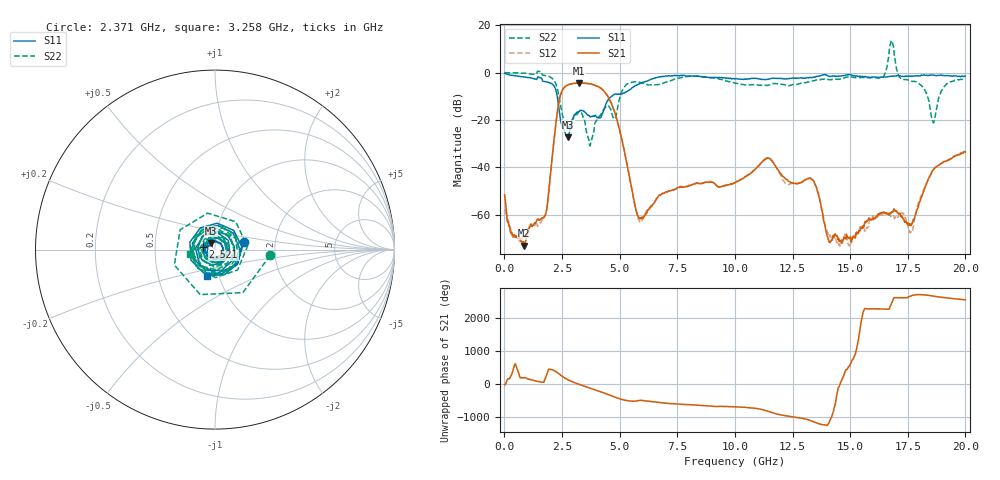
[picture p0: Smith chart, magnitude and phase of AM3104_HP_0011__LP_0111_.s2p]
!Created with skrf (http://scikit-rf.org).
# Hz S RI R 50.0
!freq ReS11 ImS11 ReS21 ImS21 ReS12 ImS12 ReS22 ImS22
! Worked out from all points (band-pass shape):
!   1601 points, 10 MHz to 20 GHz, reference 50 ohm
!   highest |S21| = -4.39 dB at 3.246 GHz (marker M1); lowest = -73.2 dB at 859.6 MHz (marker M2)
!   |S21| within 3 dB of the highest: 2.516 GHz to 4.278 GHz (1.762 GHz wide, 51.9 % of centre)
!   lowest |S11| = -27.3 dB at 2.746 GHz (marker M3), VSWR 1.09, Z = 47.7 + j3.49 ohm
!   |S11| at or under -10 dB: 2.293 GHz to 4.651 GHz (2.358 GHz wide, 67.9 % of centre)
!   |S22| runs from -31.0 to 13.6 dB; largest |S21 - S12| = 0.037
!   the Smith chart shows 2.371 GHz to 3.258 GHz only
!   S11 on the Smith chart (normalised r, x): 2.371 GHz: 1.38, +0.12; 2.521 GHz: 0.87, +0.02; 3.258 GHz: 0.88, -0.26
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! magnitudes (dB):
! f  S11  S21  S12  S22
! 10 MHz  -0.3  -51.7  -57.6  0.0
! 859.6 MHz  -1.9  -73.2  -69.1  -0.2
! 1.784 GHz  -3.8  -60.0  -60.2  -1.3
! 2.371 GHz  -15.6  -12.2  -12.2  -10.2
! 2.521 GHz  -23.3  -7.3  -7.3  -18.0
! 2.746 GHz  -27.3  -5.2  -5.2  -23.6
! 3.246 GHz  -16.5  -4.4  -4.5  -17.0
! 3.258 GHz  -16.3  -4.4  -4.5  -17.1
! 3.346 GHz  -16.0  -4.4  -4.5  -17.1
! 3.721 GHz  -18.7  -4.7  -4.8  -30.8
! 4.658 GHz  -9.9  -13.4  -13.5  -17.2
! 5.845 GHz  -4.9  -61.5  -62.6  -4.0
! 6.682 GHz  -1.9  -52.4  -52.5  -5.1
! 10.01 GHz  -2.7  -46.6  -46.6  -4.5
! 11.43 GHz  -2.8  -36.0  -36.2  -5.4
! 13.34 GHz  -2.1  -45.1  -45.2  -3.6
! 14.13 GHz  -1.6  -71.9  -68.8  -3.0
! 16.36 GHz  -1.9  -59.3  -60.1  -2.3
! 16.68 GHz  -1.6  -60.3  -60.3  7.2
! 17.65 GHz  -1.5  -64.4  -66.7  -3.6
! 18.6 GHz  -1.1  -41.2  -41.5  -21.1
! 20 GHz  -1.5  -33.6  -32.9  -2.5
